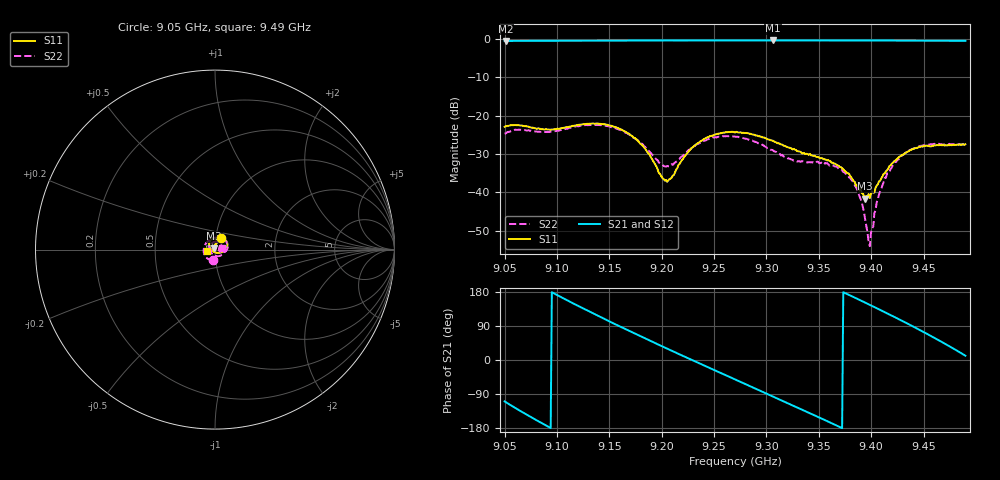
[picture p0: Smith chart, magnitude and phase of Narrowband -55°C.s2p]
!Agilent Technologies,N5230C,MY49001174,A.09.42.22
!Agilent N5230C: A.09.42.22
!Date: Friday, February 13, 2026 11:53:25
!Correction: S11(Full 2 Port(1,2))
!S21(Full 2 Port(1,2))
!S12(Full 2 Port(1,2))
!S22(Full 2 Port(1,2))
!S2P File: Measurements: S11, S21, S12, S22:
# Hz S  dB  R 50
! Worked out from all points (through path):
!   401 points, 9.05 GHz to 9.49 GHz, reference 50 ohm
!   highest |S21| = -0.35 dB at 9.3063 GHz (marker M1); lowest = -0.5 dB at 9.0511 GHz (marker M2)
!   lowest |S11| = -41.6 dB at 9.3943 GHz (marker M3), VSWR 1.02, Z = 49.5 + j0.66 ohm
!   |S11| at or under -10 dB: start of sweep to end of sweep
!   |S22| runs from -54.1 to -22.3 dB; largest |S21 - S12| = 0.0021
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9.05e9  -22.90 61.9  -0.48 -109.3  -0.48 -109.3  -24.68 -101.7
9.0511e9  -22.78 62.0  -0.48 -111.2  -0.48 -111.2  -24.62 -105.7
9.0863e9  -23.55 53.3  -0.43 -167.8  -0.43 -167.9  -24.25 151.8
9.1039e9  -23.28 54.5  -0.42 166.0  -0.42 166.0  -23.76 99.6
9.1237e9  -22.30 46.6  -0.41 137.7  -0.41 137.8  -22.54 53.9
9.16e9  -23.43 10.4  -0.39 88.5  -0.39 88.5  -23.69 -2.5
9.182e9  -27.88 -22.7  -0.36 59.8  -0.37 59.8  -27.53 -21.5
9.1974e9  -35.01 -65.9  -0.36 39.9  -0.36 40.0  -32.25 -13.9
9.2073e9  -36.58 -137.0  -0.36 27.3  -0.36 27.3  -33.23 10.9
9.2326e9  -27.61 140.3  -0.35 -4.6  -0.36 -4.6  -27.57 26.8
9.27e9  -24.40 97.6  -0.36 -51.1  -0.36 -51.1  -25.46 -15.3
9.3063e9  -26.57 76.8  -0.35 -96.2  -0.36 -96.2  -29.04 -85.4
9.3437e9  -30.40 82.1  -0.35 -143.1  -0.35 -143.1  -32.22 160.6
9.3789e9  -35.17 90.2  -0.37 171.7  -0.36 171.7  -36.10 79.8
9.3877e9  -38.82 105.1  -0.37 160.1  -0.35 160.1  -40.08 56.6
9.3943e9  -41.64 126.4  -0.37 151.4  -0.36 151.5  -47.12 27.6
9.3965e9  -41.27 139.2  -0.37 148.5  -0.37 148.4  -50.49 -3.7
9.3998e9  -40.39 158.6  -0.37 144.1  -0.37 144.1  -50.66 -60.6
9.4075e9  -37.13 -179.9  -0.37 133.7  -0.37 133.7  -40.59 -134.1
9.4174e9  -33.19 -169.2  -0.38 120.2  -0.37 120.2  -34.88 -158.6
9.4526e9  -27.81 -175.2  -0.41 70.1  -0.40 70.1  -27.56 123.1
9.49e9  -27.49 -172.5  -0.45 11.3  -0.45 11.3  -27.62 14.2
